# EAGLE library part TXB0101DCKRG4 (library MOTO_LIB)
1 bit logic level shifter
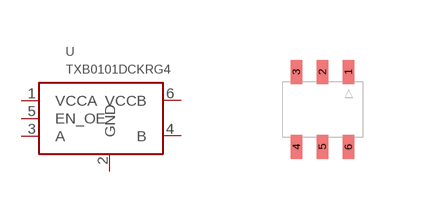
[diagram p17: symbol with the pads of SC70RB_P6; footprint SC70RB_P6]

Designator prefix U

## TXB0101DCKRG4 (MPN: TXB0101DCKRG4; SUPPLIER: TI)  [SC70RB_P6]
1  VCCA
2  GND
3  A
4  B
5  EN_OE
6  VCCB

## Footprint SC70RB_P6 (pad centres in mm)
smd 0.28 x 0.6: 1 0.65,0.94; 2 0,0.94; 3 -0.65,0.94; 4 -0.65,-0.94; 5 0,-0.94; 6 0.65,-0.94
